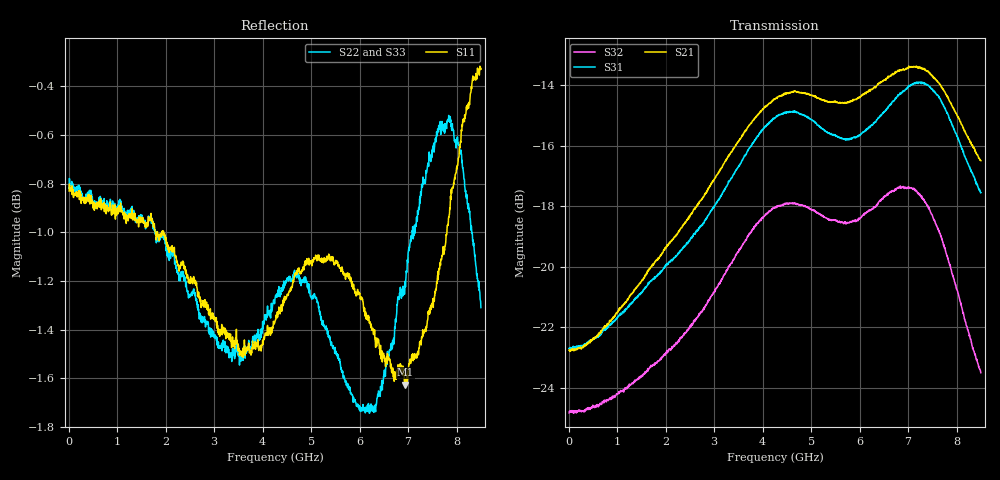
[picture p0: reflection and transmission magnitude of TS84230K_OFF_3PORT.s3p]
! Created with skrf (http://scikit-rf.org).
# Hz S RI R 50.0
!freq ReS11 ImS11 ReS12 ImS12 ReS13 ImS13
! ReS21 ImS21 ReS22 ImS22 ReS23 ImS23
! ReS31 ImS31 ReS32 ImS32 ReS33 ImS33
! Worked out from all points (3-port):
!   1601 points, 10 MHz to 8.5 GHz, reference 50 ohm
!   strongest paths, dB at 10 MHz, 2.132 GHz, 4.255 GHz, 6.378 GHz, 8.5 GHz:
!     S21: -22.8, -19.1, -14.5, -14.0, -16.5
!     S31: -22.7, -19.8, -15.1, -15.1, -17.6
!     S32: -24.8, -22.6, -18.0, -17.9, -23.5
!   lowest |S11| = -1.6 dB at 6.945 GHz (marker M1), VSWR 10.72, Z = 19.7 + j88.1 ohm
!   |S11| at or under -10 dB: nowhere
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1e7  -0.9089 0.0031  0.0727 -0.000125  0.0734 -0.000204
     0.0728 -0.000286  -0.91 0.00455  0.0575 -0.000158
     0.0733 0.000132  0.0573 3.98e-05  -0.9126 0.00463
2.392506e9  -0.671 0.5636  0.1183 0.00325  0.1083 -0.00339
            0.1179 0.00325  -0.5334 0.6902  0.0752 -0.0185
            0.1081 -0.00324  0.0753 -0.0188  -0.5361 0.6911
3.315794e9  -0.4858 0.6957  0.1509 -0.0259  0.1361 -0.0262
            0.1508 -0.0257  -0.1992 0.816  0.0889 -0.0459
            0.1359 -0.026  0.0892 -0.0455  -0.2527 0.8108
4.255e9  -0.1576 0.8398  0.162 -0.0987  0.1487 -0.0951
         0.1618 -0.0984  0.3051 0.808  0.0733 -0.1018
         0.1488 -0.0946  0.0737 -0.1016  0.2505 0.8191
4.971344e9  0.1077 0.8721  0.1244 -0.1467  0.1073 -0.1397
            0.1247 -0.1468  0.5789 0.6455  0.0283 -0.1216
            0.107 -0.1394  0.0289 -0.1213  0.5907 0.6306
5.772588e9  0.2557 0.8356  0.0852 -0.1665  0.0706 -0.1462
            0.0853 -0.1662  0.7381 0.374  -0.00815 -0.1178
            0.0707 -0.146  -0.00792 -0.1179  0.7408 0.4077
6.414644e9  0.3316 0.7762  0.0563 -0.1935  0.055 -0.1689
            0.0563 -0.1936  0.8246 0.0216  -0.0403 -0.1221
            0.0551 -0.1686  -0.0405 -0.122  0.821 0.1744
6.945269e9  0.4476 0.6982  0.00653 -0.2121  0.0137 -0.1956
            0.00648 -0.212  0.7993 -0.34  -0.0856 -0.1047
            0.014 -0.1959  -0.0852 -0.1046  0.8356 -0.1946
7.751819e9  0.733 0.4936  -0.0792 -0.1778  -0.0795 -0.1652
            -0.0792 -0.1778  0.5678 -0.7417  -0.1043 -0.0265
            -0.0787 -0.1651  -0.1039 -0.0264  0.5539 -0.7457
8.5e9  0.9276 0.258  -0.0983 -0.1128  -0.0904 -0.0971
       -0.098 -0.1132  0.344 -0.7883  -0.067 0.00308
       -0.0901 -0.0973  -0.0667 0.00298  0.3552 -0.7975
